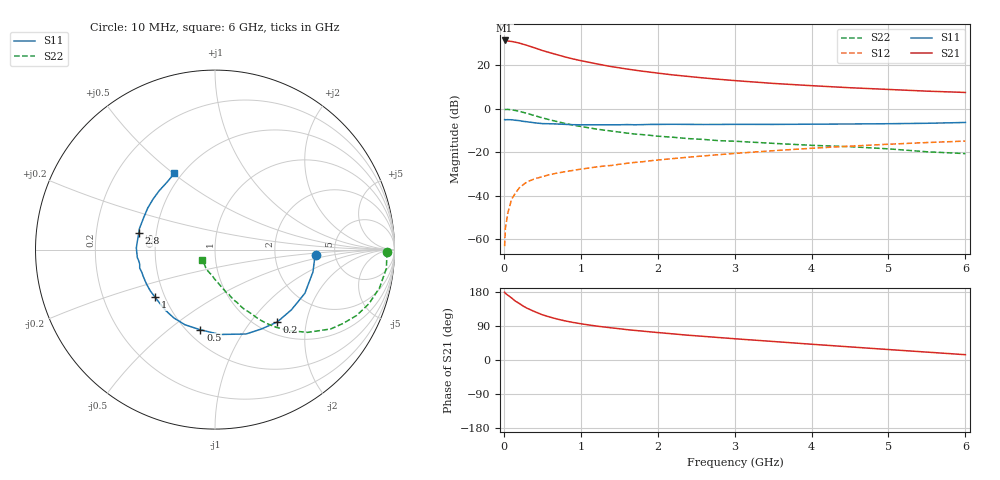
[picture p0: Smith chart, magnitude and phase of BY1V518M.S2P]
! SIEMENS Small Signal Semiconductors
! BFY420
! Si NPN RF SIEGET Grounded Emitter Transistor in MICRO-X
! VCE = 1.5 V  IC = 18 mA
! Common Emitter S-Parameters:  October  1996
# GHz  S  MA  R  50
!  f  S11  S21  S12  S22
! GHz  MAG  ANG  MAG  ANG  MAG  ANG  MAG  ANG
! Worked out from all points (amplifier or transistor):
!   36 points, 10 MHz to 6 GHz, reference 50 ohm
!   highest |S21| = 31.3 dB at 10 MHz (marker M1)
!   |S21| within 3 dB of that: start of sweep to 365.8 MHz
!   unconditionally stable (mu >= 1): start of sweep to 10.74 MHz; 1.98 GHz to end of sweep
!   at 250 MHz: K = 0.28, MSG = 32.3 dB, |S12| = -34.9 dB
!   at 1.4 GHz: K = 0.91, MSG = 22.7 dB, |S12| = -26.1 dB
!   at 6 GHz: K = 1.09, MAG = 9.4 dB, |S12| = -14.9 dB
!   S11 on the Smith chart (normalised r, x): 10 MHz: 3.53, -0.29; 200 MHz: 1.22, -1.37; 500 MHz: 0.58, -0.65; 1 GHz: 0.44, -0.29; 2.8 GHz: 0.40, +0.09; 6 GHz: 0.46, +0.51
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0.01  0.5615 -2.9  36.75 178.8  0.0007 87.7  0.9579 -0.8
0.02  0.5573 -5.8  36.48 175.9  0.0018 87.8  0.958 -2.1
0.1  0.5567 -25.9  34.93 163.9  0.0083 82.8  0.9411 -13.1
0.15  0.5421 -38.2  33.49 155.4  0.0115 74.1  0.9089 -19.4
0.2  0.5319 -49.3  32.02 149.3  0.0152 70.8  0.8707 -24.9
0.25  0.5121 -59.9  30.16 142.5  0.0179 67.6  0.8233 -30.0
0.3  0.501 -69.8  28.36 136.8  0.0208 64.9  0.7822 -34.4
0.4  0.4737 -86.6  24.88 127.7  0.0246 60.5  0.692 -41.8
0.5  0.4543 -100.3  21.64 119.4  0.0275 57.2  0.6157 -47.2
0.6  0.451 -111.7  19.22 113.2  0.0308 56.5  0.5535 -51.6
0.7  0.4445 -121.1  17.16 107.7  0.0335 54.7  0.5012 -55.1
0.8  0.4365 -129.2  15.31 103.1  0.0359 54.0  0.4565 -57.9
1  0.4263 -141.6  12.64 95.7  0.0409 54.5  0.391 -61.9
1.1  0.4276 -147.5  11.67 92.6  0.0433 54.4  0.3651 -64.3
1.4  0.4267 -159.6  9.217 84.8  0.0498 54.6  0.3069 -68.7
1.6  0.4318 -166.2  8.121 80.1  0.0559 54.2  0.2753 -71.6
2.2  0.4384 178.9  5.946 68.9  0.0716 52.8  0.2209 -78.7
2.8  0.4348 167.5  4.718 59.2  0.0882 50.1  0.1844 -85.0
3.5  0.4355 155.9  3.801 48.9  0.1084 45.7  0.1602 -92.0
4.5  0.4452 140.9  3.024 34.6  0.1381 37.6  0.1343 -102.4
5.5  0.4622 124.8  2.524 20.8  0.167 28.2  0.1026 -124.3
6  0.4824 117.9  2.356 14.0  0.1804 23.4  0.0931 -141.1
